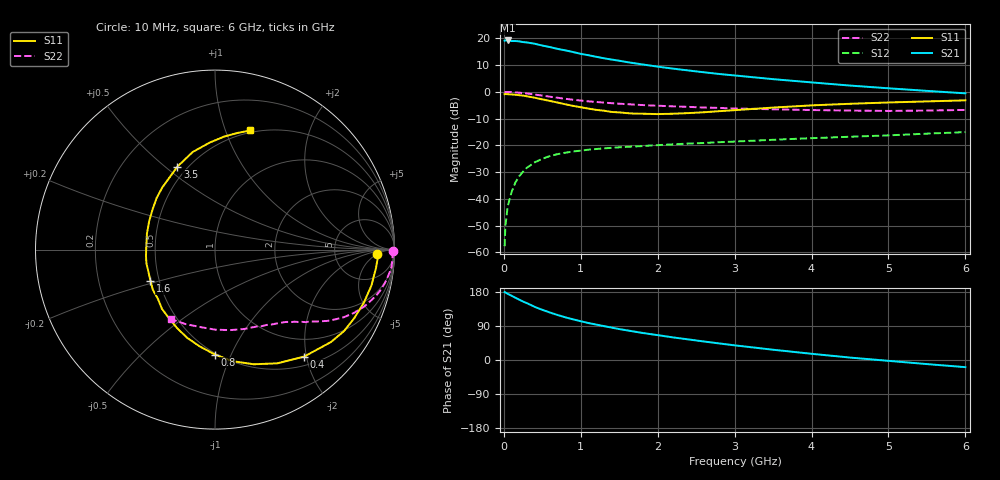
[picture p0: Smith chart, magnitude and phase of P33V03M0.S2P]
! SIEMENS Small Signal Semiconductors
! BFP181
! Si NPN RF Bipolar Junction Transistor in SOT143
! VCE = 3 V  IC = 3 mA
! Common Emitter S-Parameters:  March  1996
# GHz  S  MA  R  50
!  f  S11  S21  S12  S22
! GHz  MAG  ANG  MAG  ANG  MAG  ANG  MAG  ANG
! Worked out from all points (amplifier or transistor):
!   36 points, 10 MHz to 6 GHz, reference 50 ohm
!   highest |S21| = 19.2 dB at 50 MHz (marker M1)
!   |S21| within 3 dB of that: start of sweep to 676.1 MHz
!   unconditionally stable (mu >= 1): 2.09 GHz to end of sweep
!   at 250 MHz: K = 0.15, MSG = 24.2 dB, |S12| = -29.8 dB
!   at 1.4 GHz: K = 0.77, MSG = 16.5 dB, |S12| = -21.0 dB
!   at 6 GHz: K = 1.09, MAG = 5.4 dB, |S12| = -15.1 dB
!   lowest NFmin = 1.40 dB at 450 MHz
!   S11 on the Smith chart (normalised r, x): 10 MHz: 18, -5; 400 MHz: 0.65, -1.96; 800 MHz: 0.49, -0.87; 1.6 GHz: 0.45, -0.19; 3.5 GHz: 0.44, +0.55; 6 GHz: 0.48, +1.22
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0.01  0.9031 -1.7  9.042 179.0  0.0013 88.7  0.9941 -0.6
0.02  0.9087 -2.6  9.126 178.3  0.0031 91.0  0.9871 -1.1
0.05  0.903 -6.4  9.127 174.8  0.0072 90.0  0.9913 -3.0
0.1  0.8942 -13.0  8.905 169.7  0.0133 81.8  0.9875 -5.9
0.2  0.8648 -26.2  8.779 159.2  0.0263 74.4  0.9633 -11.4
0.3  0.8262 -38.6  8.38 150.0  0.0381 68.3  0.9301 -16.4
0.4  0.7757 -50.2  7.93 140.4  0.0479 62.3  0.8908 -20.8
0.5  0.723 -61.2  7.329 132.4  0.056 56.6  0.8495 -24.6
0.6  0.6745 -71.3  6.863 125.3  0.063 52.4  0.8105 -27.7
0.7  0.6295 -81.0  6.34 118.6  0.0684 48.7  0.7739 -30.2
0.8  0.5846 -90.0  5.956 112.6  0.0727 45.6  0.7414 -32.4
1  0.5152 -107.6  5.129 102.3  0.0794 40.4  0.6855 -35.8
1.1  0.4848 -116.0  4.834 97.5  0.0829 38.3  0.6635 -37.2
1.3  0.4435 -131.7  4.242 89.4  0.0877 35.4  0.6288 -39.8
1.6  0.3996 -154.1  3.6 78.3  0.0937 32.6  0.589 -43.2
1.8  0.3897 -168.5  3.253 71.5  0.0966 31.3  0.5659 -45.4
2.2  0.3895 166.9  2.713 59.6  0.1042 29.1  0.5348 -50.3
2.8  0.4343 138.4  2.154 43.7  0.1143 26.4  0.4999 -58.6
3.5  0.5074 114.4  1.725 27.1  0.1268 23.9  0.4713 -69.9
4.5  0.5971 92.8  1.309 6.4  0.1445 19.3  0.4461 -89.9
5.5  0.6618 79.1  1.041 -10.8  0.1652 15.6  0.4463 -111.6
6  0.6923 73.5  0.937 -18.9  0.1765 12.7  0.4584 -122.7
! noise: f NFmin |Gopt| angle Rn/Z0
0.45  1.4  0.56  17  0.36
0.9  1.5  0.45  35  0.34
1.8  1.85  0.25  82  0.36
